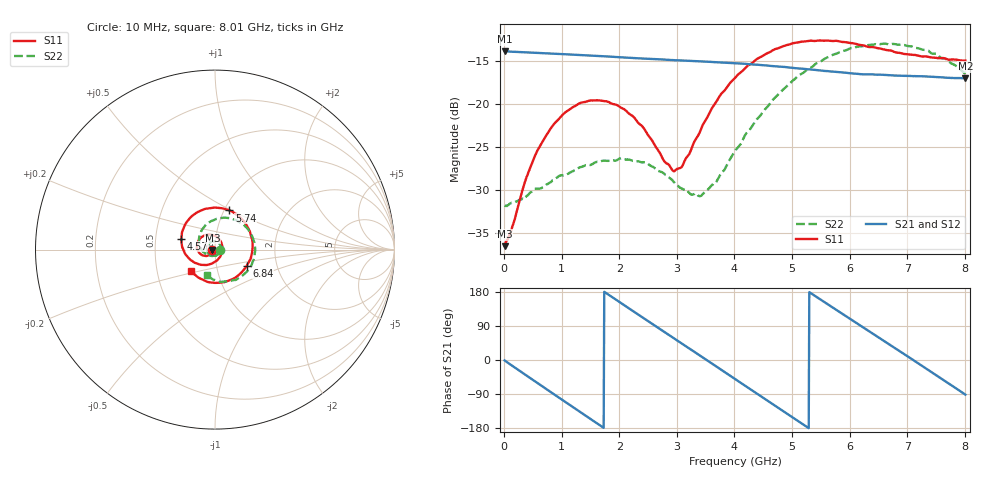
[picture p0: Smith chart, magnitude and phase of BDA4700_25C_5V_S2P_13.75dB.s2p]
!Agilent Technologies,E5071B,MY42404982,A.09.10
!Date: Mon Oct 20 13:33:03 2025
!Data & Calibration Information:
!Freq	S11:SOLT2(ON)	S21:SOLT2(ON)	S12:SOLT2(ON)	S22:SOLT2(ON)
# Hz S RI R 50
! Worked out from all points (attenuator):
!   801 points, 10 MHz to 8.01 GHz, reference 50 ohm
!   highest |S21| = -13.86 dB at 10 MHz (marker M1); lowest = -17.0 dB at 8.01 GHz (marker M2)
!   lowest |S11| = -36.5 dB at 10 MHz (marker M3), VSWR 1.03, Z = 48.5 - j0.137 ohm
!   |S11| at or under -10 dB: start of sweep to end of sweep
!   |S22| runs from -31.8 to -13.0 dB; largest |S21 - S12| = 0.0015
!   S11 on the Smith chart (normalised r, x): 10 MHz: 0.97, -0.00; 4.57 GHz: 0.68, +0.09; 5.74 GHz: 1.06, +0.49; 6.84 GHz: 1.40, -0.26; 8.01 GHz: 0.75, -0.18
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1e7  -0.0149 -0.00141  0.2028 -0.00445  0.2027 -0.00462  0.0257 -0.000991
3.9e8  -0.0265 -0.0267  0.1504 -0.131  0.1504 -0.1311  0.0207 -0.0206
6e8  -0.0426 -0.0351  0.0905 -0.1761  0.0904 -0.1761  0.0121 -0.0299
1e9  -0.082 -0.0237  -0.0475 -0.1891  -0.0475 -0.1893  -0.0176 -0.0344
1.35e9  -0.1012 0.0128  -0.1476 -0.1235  -0.1477 -0.1235  -0.0405 -0.0151
1.71e9  -0.0863 0.0583  -0.1892 -0.01  -0.1893 -0.00987  -0.0441 0.0158
2.08e9  -0.0413 0.084  -0.1532 0.1063  -0.1533 0.1063  -0.0242 0.0413
2.68e9  0.0342 0.0412  0.0174 0.1811  0.0175 0.181  0.0238 0.0333
2.93e9  0.0411 0.00105  0.0921 0.1547  0.0921 0.1544  0.0324 0.0153
3.07e9  0.0363 -0.0225  0.1266 0.1268  0.126 0.1272  0.0324 0.00265
3.43e9  -0.00734 -0.0725  0.1748 0.0269  0.1749 0.0268  0.0155 -0.0251
3.69e9  -0.0583 -0.0857  0.1668 -0.0526  0.1668 -0.053  -0.0082 -0.0345
4.01e9  -0.1263 -0.0642  0.111 -0.1324  0.1111 -0.1323  -0.0445 -0.029
4.57e9  -0.1875 0.0607  -0.049 -0.16  -0.0489 -0.1601  -0.088 0.0391
4.98e9  -0.1437 0.1708  -0.1386 -0.0849  -0.1389 -0.0853  -0.0706 0.1136
5.35e9  -0.0462 0.2282  -0.1576 0.0163  -0.1577 0.0158  -0.00678 0.1642
5.74e9  0.0808 0.2182  -0.1091 0.1086  -0.109 0.1086  0.0885 0.1735
6.22e9  0.1908 0.1087  0.0057 0.1487  0.00707 0.149  0.1929 0.0991
6.68e9  0.2009 -0.0413  0.1092 0.0985  0.1095 0.0983  0.2211 -0.0241
6.84e9  0.1775 -0.0893  0.1311 0.0646  0.1315 0.0637  0.2101 -0.0674
7.42e9  0.0254 -0.1847  0.1225 -0.0761  0.1224 -0.0763  0.0976 -0.1711
8.01e9  -0.1329 -0.1195  -0.00342 -0.141  -0.0032 -0.1412  -0.0464 -0.1422
